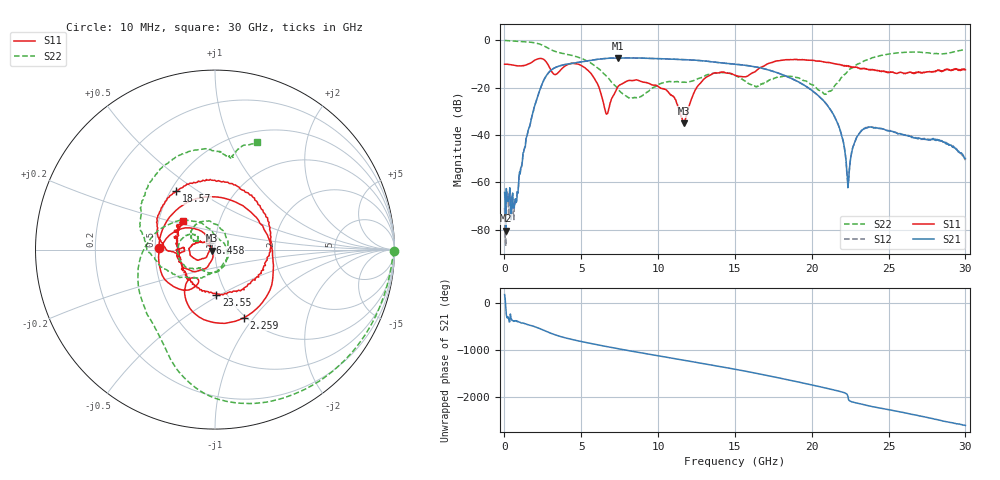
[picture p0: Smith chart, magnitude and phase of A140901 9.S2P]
!  2-Port S-parameters saved by WinCal
! VAR MeasName=S-Parameters (CALIBRATED_DATA) read from VNA (N5244A)
! VAR MeasDate=11/3/2014 9:27:29 AM
! VAR NAME=A140901 9
! VAR FILENAME=A140901 9.S2P
! VAR DATE=11/3/2014 9:27:29 AM
! VAR PHYS_PORTS=1,2
# Hz S RI R 50
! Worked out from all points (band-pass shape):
!   801 points, 10 MHz to 30 GHz, reference 50 ohm
!   highest |S21| = -7.42 dB at 7.395 GHz (marker M1); lowest = -80.5 dB at 84.97 MHz (marker M2)
!   |S21| within 3 dB of the highest: 3.789 GHz to 15.51 GHz (11.72 GHz wide, 121 % of centre)
!   lowest |S11| = -35.0 dB at 11.71 GHz (marker M3), VSWR 1.04, Z = 48.4 - j0.632 ohm
!   |S11| at or under -10 dB: start of sweep to 1.543 GHz; 4.763 GHz to 17.1 GHz (12.33 GHz wide, 113 % of centre); 21.64 GHz to end of sweep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
!   |S22| runs from -24.5 to 0.0 dB; largest |S21 - S12| = 0.0026
!   S11 on the Smith chart (normalised r, x): 10 MHz: 0.52, +0.01; 2.259 GHz: 0.98, -0.90; 6.458 GHz: 0.94, +0.07; 18.57 GHz: 0.53, +0.41; 23.55 GHz: 0.89, -0.48; 30 GHz: 0.67, +0.23
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1e7  -0.3122 0.00668  -0.000607 3.97e-06  0.000126 -0.000257  0.9958 -0.00774
8.4975e7  -0.308 0.0603  -7.89e-07 -9.44e-05  2.87e-05 -3.4e-05  0.9872 -0.0615
7.222625e8  0.013 0.2929  0.00043 -0.00012  0.000397 -0.000183  0.8615 -0.4337
2.25925e9  0.1618 -0.3791  -0.0814 -0.000679  -0.0812 -0.000604  0.0423 -0.8403
3.796238e9  -0.1408 -0.2228  0.2996 -0.0353  0.2988 -0.0353  -0.3619 -0.3855
5.033325e9  -0.2869 0.0388  -0.0711 -0.3465  -0.071 -0.3461  -0.4117 -0.0358
6.45785e9  -0.0296 0.0347  -0.3971 0.1042  -0.3972 0.1034  -0.1204 0.1574
7.395038e9  -0.0892 -0.0575  -0.1241 0.407  -0.1249 0.4068  -0.0108 0.0925
8.819562e9  -0.1372 0.0135  0.3872 0.1692  0.387 0.1688  0.0636 0.0011
1.001916e10  -0.0988 0.0384  0.2961 -0.2856  0.2951 -0.2856  0.0289 -0.1118
1.17061e10  -0.0165 -0.00653  -0.2946 -0.2593  -0.2947 -0.2595  -0.079 -0.1038
1.305565e10  -0.1033 -0.1215  -0.2962 0.2167  -0.295 0.217  -0.1444 -0.1042
1.5005e10  -0.1828 0.0107  0.2674 0.1625  0.2673 0.1618  -0.1644 0.0755
1.669194e10  -0.2684 -0.0037  0.067 -0.2528  0.0652 -0.2536  -0.1102 0.0482
1.856631e10  -0.2176 0.3244  -0.1503 0.0595  -0.1502 0.0589  -0.0837 0.1502
2.002832e10  0.096 0.3677  0.0486 0.0714  0.048 0.0717  0.0461 0.1052
2.164029e10  0.3144 0.0404  0.00803 -0.017  0.00821 -0.0172  0.00407 -0.1223
2.235255e10  0.2558 -0.1321  -0.000762 6.94e-05  -0.000918 0.000208  -0.1625 -0.1528
2.283989e10  0.1615 -0.2243  0.00584 0.00482  0.00579 0.00501  -0.2685 -0.1127
2.355215e10  0.00727 -0.2517  0.0136 -0.00374  0.0138 -0.00389  -0.38 0.0111
2.501416e10  -0.1674 -0.1214  -0.00389 -0.0116  -0.00385 -0.0116  -0.372 0.356
3e10  -0.1787 0.1602  0.000317 -0.00316  0.000335 -0.00291  0.2339 0.5986
